PROGRAM MAIN
VAR
	myDebug : BOOL;
	ChangeTo1 : BOOL;
	ChangeTo2 : BOOL;
END_VAR

IF myFanControl.IsOn THEN
	myDebug := TRUE;
ELSE 
	myDebug := FALSE;
END_IF

IF ChangeTo1 THEN
	ChangeTo1 := FALSE;
	myFanControlDigitalInput.ChangeDigitalInput(device1.GetDigitalInput(0));
END_IF

IF ChangeTo2 THEN
	ChangeTo2 := FALSE;
	myFanControlDigitalInput.ChangeDigitalInput(device1.GetDigitalInput(1));
END_IF

END_PROGRAM
